TYPE IDENTControl_UserData :
STRUCT	
	ReadData:			ARRAY[0..245] OF BYTE;	(* Read in data from data carrier*)	
	WriteData:			ARRAY[0..245] OF BYTE;	(* Write data to data carrier *)
	SpecialCommand:		ARRAY[0..30] OF BYTE;	(* Bypass for commands, which are not included in FB *)
END_STRUCT
END_TYPE
